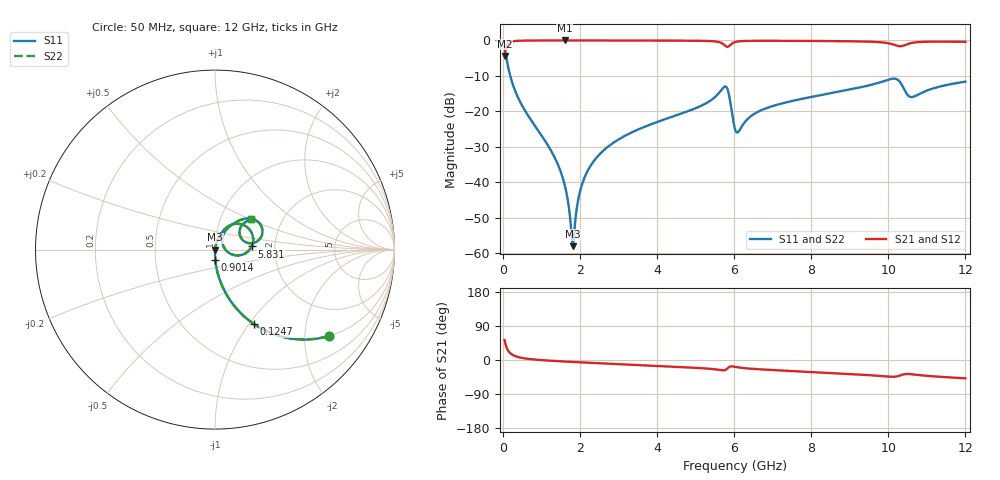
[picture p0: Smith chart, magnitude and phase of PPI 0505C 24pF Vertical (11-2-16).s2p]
# GHz S MA R 50
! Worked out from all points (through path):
!   1601 points, 50 MHz to 12 GHz, reference 50 ohm
!   highest |S21| = -0.01 dB at 1.611 GHz (marker M1); lowest = -4.4 dB at 50 MHz (marker M2)
!   group delay of S21, straight-line fit = 12.6 ps
!   lowest |S11| = -58.0 dB at 1.82 GHz (marker M3), VSWR 1.00, Z = 50.1 - j0.00542 ohm
!   |S11| at or under -10 dB: 196.1 MHz to end of sweep
!   |S22| runs from -58.0 to -2.0 dB; largest |S21 - S12| = 0
!   S11 on the Smith chart (normalised r, x): 50 MHz: 0.99, -2.64; 124.7 MHz: 0.99, -1.05; 901.4 MHz: 1.00, -0.11; 5.831 GHz: 1.51, +0.06; 12 GHz: 1.40, +0.50
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0.05  0.7974 -37.2  0.6032 52.7  0.6032 52.7  0.7974 -37.2
0.1246875  0.4668 -62.5  0.884 27.5  0.884 27.5  0.4668 -62.5
0.2143125  0.2911 -73.6  0.9562 16.3  0.9562 16.3  0.2911 -73.6
0.3860938  0.1615 -81.6  0.9862 8.2  0.9862 8.2  0.1615 -81.6
0.9014375  0.05547 -88.4  0.9975 0.6  0.9975 0.6  0.05547 -88.4
1.357031  0.02182 -89.7  0.9986 -2.6  0.9986 -2.6  0.02182 -89.7
1.610969  0.009036 -86.5  0.9987 -4.1  0.9987 -4.1  0.009036 -86.5
1.820094  0.001256 -2.5  0.9986 -5.2  0.9986 -5.2  0.001256 -2.5
2.044156  0.008813 75.0  0.9985 -6.3  0.9985 -6.3  0.008813 75.0
2.290625  0.01747 77.9  0.9983 -7.5  0.9983 -7.5  0.01747 77.9
2.671531  0.02986 77.8  0.9979 -9.3  0.9979 -9.3  0.02986 77.8
4.038312  0.07183 72.7  0.995 -15.6  0.995 -15.6  0.07183 72.7
5.636625  0.1891 49.6  0.9372 -26.5  0.9372 -26.5  0.1891 49.6
5.830813  0.2053 5.0  0.812 -21.8  0.812 -21.8  0.2053 5.0
6.025  0.05626 2.2  0.9467 -18.1  0.9467 -18.1  0.05626 2.2
6.107156  0.05113 31.8  0.9669 -19.5  0.9669 -19.5  0.05113 31.8
6.779344  0.1078 61.4  0.9875 -25.3  0.9875 -25.3  0.1078 61.4
8.019156  0.1602 56.7  0.9822 -31.7  0.9822 -31.7  0.1602 56.7
10.01331  0.2803 35.7  0.9098 -43.9  0.9098 -43.9  0.2803 35.7
10.25231  0.2772 18.4  0.8349 -42.6  0.8349 -42.6  0.2772 18.4
10.60334  0.1588 26.4  0.9196 -37.7  0.9196 -37.7  0.1588 26.4
12  0.2624 39.9  0.9561 -48.4  0.9561 -48.4  0.2624 39.9
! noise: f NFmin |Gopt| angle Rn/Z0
0.05  0.0003849  0.8642  0.958  0.0006084
1.372  0.003933  0.6704  4.004  0.002292
2.701  0.006561  0.6227  7.476  0.003236
4.031  0.00947  0.6133  10.93  0.00451
5.36  0.02391  0.7765  14.89  0.02151
6.682  0.02172  0.7066  18.45  0.01418
8.012  0.0192  0.6237  21.41  0.009224
9.341  0.02995  0.7062  25.27  0.0191
10.67  0.07721  0.8588  29.53  0.1095
12  0.03184  0.6597  31.77  0.0166
